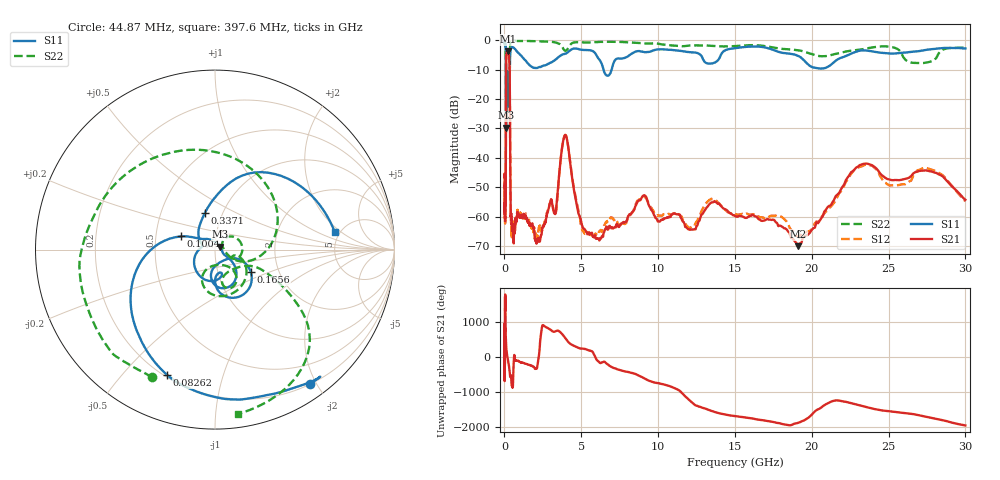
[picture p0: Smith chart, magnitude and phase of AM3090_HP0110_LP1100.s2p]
! Date/Time: Thu, Feb 28, 2019 2:00 PM
! Network Analyzer: Agilent Technologies E8364B Rev: A.07.50.67
! Sweep from 0.010 to 30.000 GHz, 1601 Points, Sweep Type: LOG
! Power Supply: 5.023 V, 0.002 A
# Hz S DB R 50
!freq MagS11 AngS11 MagS21 AngS21 MagS12 AngS12 MagS22 AngS22
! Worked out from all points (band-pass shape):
!   1601 points, 10 MHz to 30 GHz, reference 50 ohm
!   highest |S21| = -3.77 dB at 230.5 MHz (marker M1); lowest = -70.1 dB at 19.12 GHz (marker M2)
!   |S21| within 3 dB of the highest: 112 MHz to 320.9 MHz (208.9 MHz wide, 96.5 % of centre)
!   lowest |S11| = -29.8 dB at 107.7 MHz (marker M3), VSWR 1.07, Z = 52.8 + j1.8 ohm
!   |S11| at or under -10 dB: 98.37 MHz to 349.7 MHz (251.3 MHz wide, 112 % of centre); 6.447 GHz to 6.978 GHz (530.9 MHz wide, 7.91 % of centre)
!   |S22| runs from -26.8 to -0.1 dB; largest |S21 - S12| = 0.0097
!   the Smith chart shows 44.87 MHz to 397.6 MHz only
!   S11 on the Smith chart (normalised r, x): 44.87 MHz: 0.20, -1.92; 82.62 MHz: 0.21, -0.67; 100.4 MHz: 0.68, +0.10; 165.6 MHz: 1.44, -0.38; 337.1 MHz: 0.83, +0.35; 397.6 MHz: 4.49, +1.66
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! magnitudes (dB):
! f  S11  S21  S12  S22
! 10 MHz  -0.3  -46.5  -51.4  -0.6
! 38.04 MHz  -0.5  -60.4  -59.0  -1.5
! 44.87 MHz  -0.7  -56.4  -56.5  -2.0
! 82.62 MHz  -2.5  -51.7  -50.1  -4.7
! 100.4 MHz  -13.9  -15.3  -15.2  -13.3
! 107.7 MHz  -29.8  -8.3  -8.3  -26.2
! 122.7 MHz  -13.2  -5.3  -5.2  -17.2
! 144.7 MHz  -22.4  -4.1  -4.0  -19.5
! 165.6 MHz  -12.5  -3.8  -3.7  -14.7
! 230.5 MHz  -17.7  -3.8  -3.7  -18.6
! 337.1 MHz  -13.5  -10.1  -10.0  -8.4
! 397.6 MHz  -3.4  -56.1  -52.8  -0.7
! 550.5 MHz  -2.5  -63.3  -67.2  -0.2
! 2.084 GHz  -9.5  -69.2  -66.9  -0.4
! 3.318 GHz  -6.7  -58.8  -58.9  -0.8
! 3.953 GHz  -4.7  -32.2  -32.2  -3.6
! 5.154 GHz  -3.3  -64.1  -65.3  -0.8
! 7.926 GHz  -5.8  -61.7  -62.2  -0.7
! 13.74 GHz  -7.5  -55.1  -54.6  -2.0
! 19.12 GHz  -5.4  -70.1  -67.0  -3.5
! 23.24 GHz  -3.5  -42.3  -42.9  -3.2
! 30 GHz  -2.8  -54.3  -54.7  -2.5
